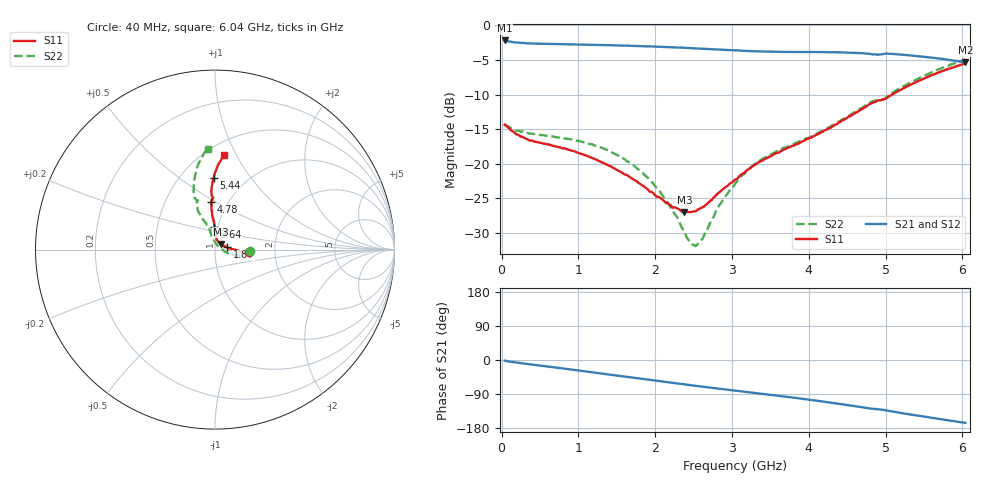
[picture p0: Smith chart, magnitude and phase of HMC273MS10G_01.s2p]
!Hittite Microwave Corporation
!12 Elizabeth Drive
!Chelmsford, MA 01824
!Tel: 978-250-3343
!Fax: 978-250-3373
!Device: HMC273MS10G,  0.7-3.7 GHz GaAs 5-bit digital attenuator in 10-lead Grounded Base surface Mount Plastic Package
!Misc: Room Temp Vdd = 5V, 1dB State.
# GHZ S DB R 50.0
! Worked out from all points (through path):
!   201 points, 40 MHz to 6.04 GHz, reference 50 ohm
!   highest |S21| = -2.17 dB at 40 MHz (marker M1); lowest = -5.3 dB at 6.04 GHz (marker M2)
!   group delay of S21, straight-line fit = 74.1 ps
!   lowest |S11| = -27.0 dB at 2.38 GHz (marker M3), VSWR 1.09, Z = 53.1 + j3.36 ohm
!   |S11| at or under -10 dB: start of sweep to 5.086 GHz
!   |S22| runs from -31.9 to -5.0 dB; largest |S21 - S12| = 0.0053
!   S11 on the Smith chart (normalised r, x): 40 MHz: 1.47, -0.04; 1.87 GHz: 1.14, +0.03; 3.64 GHz: 0.96, +0.24; 4.78 GHz: 0.83, +0.48; 5.44 GHz: 0.72, +0.68; 6.04 GHz: 0.61, +0.90
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0.04  -14.37 -3.7  -2.17 -1.6  -2.23 -1.7  -14.23 -2.5
0.19  -15.73 -8.5  -2.49 -6.6  -2.48 -6.7  -15.23 -6.6
0.37  -16.64 -6.3  -2.60 -11.2  -2.60 -11.2  -15.65 -7.3
1.06  -18.64 -1.2  -2.76 -29.2  -2.76 -29.1  -16.86 -12.3
1.57  -21.30 3.5  -2.90 -42.9  -2.90 -42.8  -19.09 -16.2
1.87  -23.40 11.1  -3.02 -50.8  -3.02 -50.7  -21.68 -16.2
2.05  -24.80 19.4  -3.08 -55.5  -3.08 -55.5  -23.77 -12.9
2.29  -26.43 35.2  -3.19 -61.8  -3.18 -61.7  -27.75 -1.4
2.38  -27.02 45.1  -3.23 -64.3  -3.22 -64.2  -29.73 10.1
2.47  -26.98 55.0  -3.28 -66.6  -3.28 -66.9  -31.57 28.5
2.53  -26.84 60.9  -3.33 -68.2  -3.32 -68.1  -31.90 47.7
2.62  -26.27 69.4  -3.37 -70.5  -3.37 -70.4  -30.79 69.2
2.8  -24.47 81.7  -3.48 -75.0  -3.48 -74.9  -26.61 93.2
3.04  -22.29 88.7  -3.60 -80.8  -3.60 -80.8  -22.93 102.0
3.31  -20.09 91.3  -3.73 -87.4  -3.74 -87.7  -19.91 105.3
3.64  -18.13 91.4  -3.82 -95.2  -3.81 -95.2  -17.89 105.8
4.06  -16.02 92.6  -3.85 -106.1  -3.85 -106.1  -15.88 109.5
4.45  -13.68 94.6  -3.90 -117.2  -3.89 -117.3  -13.51 113.0
4.78  -11.45 94.4  -4.09 -127.3  -4.07 -127.4  -11.25 112.2
5.05  -10.24 93.6  -4.09 -134.7  -4.08 -134.7  -10.05 111.2
5.44  -7.98 91.0  -4.48 -147.6  -4.46 -147.4  -7.62 105.7
6.04  -5.51 84.4  -5.33 -165.8  -5.31 -165.7  -4.97 94.2
